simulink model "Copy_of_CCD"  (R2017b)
settings: Solver=FixedStepDiscrete  StartTime=0.0  StopTime=10.0  FixedStep=0.01  RelTol=1e-3  EnableMultiTasking=on
undefined symbols (not defined in the file): ASWTYPE_FALSE, ASWTYPE_TRUE, CcCCD_DrvDiagtCnf_ms, CcCCD_DrvVoltHiVal_mV, CcCCD_DrvVoltLoVal_mV, CcCCD_KL30CVoltCnf_ms, CcCCD_KL30CVoltHiLmt_mV, CcCCD_KL30CVoltLoLmt_mV, CCD_RUNTIME_MS, Enum_CCDLSDState, Enum_UDSAreaSel
libraries: AIWAYS_Powertrain_BMS_lib x38
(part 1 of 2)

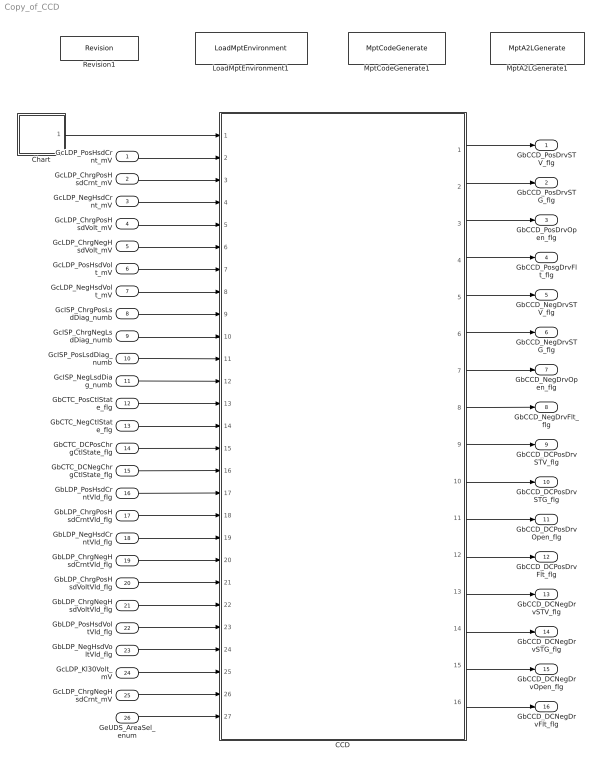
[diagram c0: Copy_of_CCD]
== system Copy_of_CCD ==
  GcLDP_PosHsdCrnt_mV : Inport
  GcLDP_ChrgPosHsdCrnt_mV : Inport  Port=2
  GcLDP_NegHsdCrnt_mV : Inport  Port=3
  GcLDP_ChrgPosHsdVolt_mV : Inport  Port=4
  GcLDP_ChrgNegHsdVolt_mV : Inport  Port=5
  GcLDP_PosHsdVolt_mV : Inport  Port=6
  GcLDP_NegHsdVolt_mV : Inport  Port=7
  GcISP_ChrgPosLsdDiag_numb : Inport  Port=8
  GcISP_ChrgNegLsdDiag_numb : Inport  Port=9
  GcISP_PosLsdDiag_numb : Inport  Port=10
  GcISP_NegLsdDiag_numb : Inport  Port=11
  GbCTC_PosCtlState_flg : Inport  Port=12
  GbCTC_NegCtlState_flg : Inport  Port=13
  GbCTC_DCPosChrgCtlState_flg : Inport  Port=14
  GbCTC_DCNegChrgCtlState_flg : Inport  Port=15
  GbLDP_PosHsdCrntVld_flg : Inport  Port=16
  GbLDP_ChrgPosHsdCrntVld_flg : Inport  Port=17
  GbLDP_NegHsdCrntVld_flg : Inport  Port=18
  GbLDP_ChrgNegHsdCrntVld_flg : Inport  Port=19
  GbLDP_ChrgPosHsdVoltVld_flg : Inport  Port=20
  GbLDP_ChrgNegHsdVoltVld_flg : Inport  Port=21
  GbLDP_PosHsdVoltVld_flg : Inport  Port=22
  GbLDP_NegHsdVoltVld_flg : Inport  Port=23
  GcLDP_Kl30Volt_mV : Inport  Port=24
  GcLDP_ChrgNegHsdCrnt_mV : Inport  Port=25
  GeUDS_AreaSel_enum : Inport  Port=26
  CCD : Subsystem
  Chart : Stateflow chart  TreatAsAtomicUnit=on
  LoadMptEnvironment1 : AIWAYS_Powertrain_BMS_lib/Config/LoadMptEnvironment  ProjectName=Comm  SuppierID=NewPlatformUAES
  MptA2LGenerate1 : AIWAYS_Powertrain_BMS_lib/Config/MptA2LGenerate  SystemSampleTime=-1
  MptCodeGenerate1 : AIWAYS_Powertrain_BMS_lib/Config/MptCodeGenerate  SystemSampleTime=-1
  Revision1 : AIWAYS_Powertrain_BMS_lib/Config/Revision  curVersion='M104C103R102'  newVersion='M104C103R102'
  GbCCD_PosDrvSTV_flg : Outport
  GbCCD_PosDrvSTG_flg : Outport  Port=2
  GbCCD_PosDrvOpen_flg : Outport  Port=3
  GbCCD_PosgDrvFlt_flg : Outport  Port=4
  GbCCD_NegDrvSTV_flg : Outport  Port=5
  GbCCD_NegDrvSTG_flg : Outport  Port=6
  GbCCD_NegDrvOpen_flg : Outport  Port=7
  GbCCD_NegDrvFlt_flg : Outport  Port=8
  GbCCD_DCPosDrvSTV_flg : Outport  Port=9
  GbCCD_DCPosDrvSTG_flg : Outport  Port=10
  GbCCD_DCPosDrvOpen_flg : Outport  Port=11
  GbCCD_DCPosDrvFlt_flg : Outport  Port=12
  GbCCD_DCNegDrvSTV_flg : Outport  Port=13
  GbCCD_DCNegDrvSTG_flg : Outport  Port=14
  GbCCD_DCNegDrvOpen_flg : Outport  Port=15
  GbCCD_DCNegDrvFlt_flg : Outport  Port=16
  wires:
  CCD/1(GbCCD_PosDrvSTV_flg) -> GbCCD_PosDrvSTV_flg/1
  CCD/2(GbCCD_PosDrvSTG_flg) -> GbCCD_PosDrvSTG_flg/1
  CCD/3(GbCCD_PosDrvOpen_flg) -> GbCCD_PosDrvOpen_flg/1
  CCD/5(GbCCD_NegDrvSTV_flg) -> GbCCD_NegDrvSTV_flg/1
  CCD/6(GbCCD_NegDrvSTG_flg) -> GbCCD_NegDrvSTG_flg/1
  CCD/7(GbCCD_NegDrvOpen_flg) -> GbCCD_NegDrvOpen_flg/1
  CCD/9(GbCCD_DCPosDrvSTV_flg) -> GbCCD_DCPosDrvSTV_flg/1
  CCD/10(GbCCD_DCPosDrvSTG_flg) -> GbCCD_DCPosDrvSTG_flg/1
  CCD/11(GbCCD_DCPosDrvOpen_flg) -> GbCCD_DCPosDrvOpen_flg/1
  CCD/13(GbCCD_DCNegDrvSTV_flg) -> GbCCD_DCNegDrvSTV_flg/1
  CCD/14(GbCCD_DCNegDrvSTG_flg) -> GbCCD_DCNegDrvSTG_flg/1
  CCD/15(GbCCD_DCNegDrvOpen_flg) -> GbCCD_DCNegDrvOpen_flg/1
  Chart/1(CCD_CoilDiag_10ms()) -> CCD/1(CCD_CoilDiag_10ms)
  GcLDP_PosHsdCrnt_mV/1 -> CCD/2(GcLDP_PosHsdCrnt_mV)
  GcLDP_ChrgPosHsdCrnt_mV/1 -> CCD/3(GcLDP_ChrgPosHsdCrnt_mV)
  GcLDP_NegHsdCrnt_mV/1 -> CCD/4(GcLDP_NegHsdCrnt_mV)
  GcLDP_ChrgPosHsdVolt_mV/1 -> CCD/5(GcLDP_ChrgPosHsdVolt_mV)
  GcLDP_ChrgNegHsdVolt_mV/1 -> CCD/6(GcLDP_ChrgNegHsdVolt_mV)
  GcLDP_PosHsdVolt_mV/1 -> CCD/7(GcLDP_PosHsdVolt_mV)
  GcLDP_NegHsdVolt_mV/1 -> CCD/8(GcLDP_NegHsdVolt_mV)
  GcISP_ChrgPosLsdDiag_numb/1 -> CCD/9(GcISP_ChrgPosLsdDiag_numb)
  GcISP_ChrgNegLsdDiag_numb/1 -> CCD/10(GcISP_ChrgNegLsdDiag_numb)
  GcISP_PosLsdDiag_numb/1 -> CCD/11(GcISP_PosLsdDiag_numb)
  GcISP_NegLsdDiag_numb/1 -> CCD/12(GcISP_NegLsdDiag_numb)
  GbCTC_PosCtlState_flg/1 -> CCD/13(GbCTC_PosCtlState_flg)
  GbCTC_NegCtlState_flg/1 -> CCD/14(GbCTC_NegCtlState_flg)
  GbCTC_DCPosChrgCtlState_flg/1 -> CCD/15(GbCTC_DCPosChrgCtlState_flg)
  GbCTC_DCNegChrgCtlState_flg/1 -> CCD/16(GbCTC_DCNegChrgCtlState_flg)
  GbLDP_PosHsdCrntVld_flg/1 -> CCD/17(GbLDP_PosHsdCrntVld_flg)
  GbLDP_ChrgPosHsdCrntVld_flg/1 -> CCD/18(GbLDP_ChrgPosHsdCrntVld_flg)
  GbLDP_NegHsdCrntVld_flg/1 -> CCD/19(GbLDP_NegHsdCrntVld_flg)
  GbLDP_ChrgNegHsdCrntVld_flg/1 -> CCD/20(GbLDP_ChrgNegHsdCrntVld_flg)
  GbLDP_ChrgPosHsdVoltVld_flg/1 -> CCD/21(GbLDP_ChrgPosHsdVoltVld_flg)
  GbLDP_ChrgNegHsdVoltVld_flg/1 -> CCD/22(GbLDP_ChrgNegHsdVoltVld_flg)
  GbLDP_PosHsdVoltVld_flg/1 -> CCD/23(GbLDP_PosHsdVoltVld_flg)
  GbLDP_NegHsdVoltVld_flg/1 -> CCD/24(GbLDP_NegHsdVoltVld_flg)
  GcLDP_Kl30Volt_mV/1 -> CCD/25(GcLDP_Kl30Volt_mV)
  GcLDP_ChrgNegHsdCrnt_mV/1 -> CCD/26(GcLDP_ChrgNegHsdCrnt_mV)
  CCD/4(GbCCD_PosgDrvFlt_flg) -> GbCCD_PosgDrvFlt_flg/1
  CCD/8(GbCCD_NegDrvFlt_flg) -> GbCCD_NegDrvFlt_flg/1
  CCD/12(GbCCD_DCPosDrvFlt_flg) -> GbCCD_DCPosDrvFlt_flg/1
  CCD/16(GbCCD_DCNegDrvFlt_flg) -> GbCCD_DCNegDrvFlt_flg/1
  GeUDS_AreaSel_enum/1 -> CCD/27(GeUDS_AreaSel_enum)

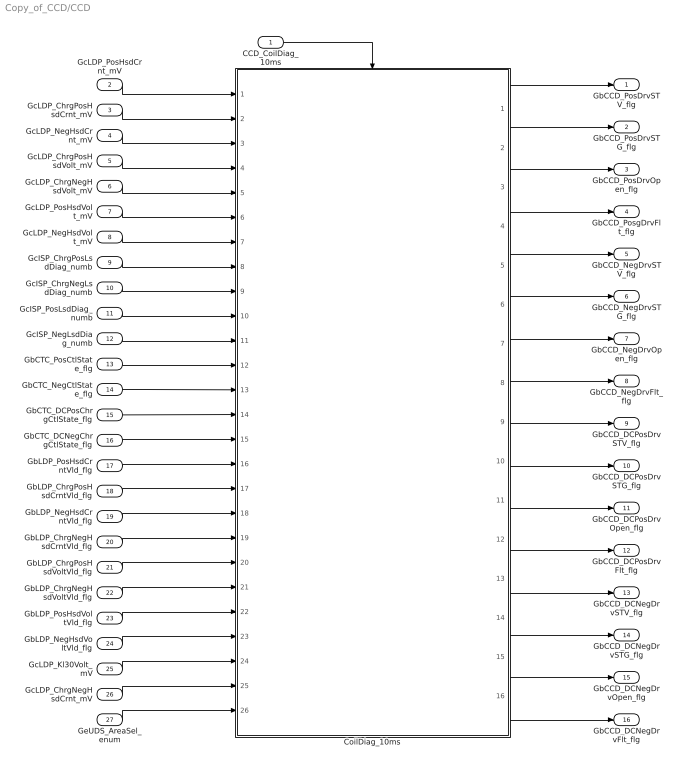
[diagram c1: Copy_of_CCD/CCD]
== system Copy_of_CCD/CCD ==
  CCD_CoilDiag_10ms : Inport
  GcLDP_PosHsdCrnt_mV : Inport  Port=2
  GcLDP_ChrgPosHsdCrnt_mV : Inport  Port=3
  GcLDP_NegHsdCrnt_mV : Inport  Port=4
  GcLDP_ChrgPosHsdVolt_mV : Inport  Port=5
  GcLDP_ChrgNegHsdVolt_mV : Inport  Port=6
  GcLDP_PosHsdVolt_mV : Inport  Port=7
  GcLDP_NegHsdVolt_mV : Inport  Port=8
  GcISP_ChrgPosLsdDiag_numb : Inport  Port=9
  GcISP_ChrgNegLsdDiag_numb : Inport  Port=10
  GcISP_PosLsdDiag_numb : Inport  Port=11
  GcISP_NegLsdDiag_numb : Inport  Port=12
  GbCTC_PosCtlState_flg : Inport  Port=13
  GbCTC_NegCtlState_flg : Inport  Port=14
  GbCTC_DCPosChrgCtlState_flg : Inport  Port=15
  GbCTC_DCNegChrgCtlState_flg : Inport  Port=16
  GbLDP_PosHsdCrntVld_flg : Inport  Port=17
  GbLDP_ChrgPosHsdCrntVld_flg : Inport  Port=18
  GbLDP_NegHsdCrntVld_flg : Inport  Port=19
  GbLDP_ChrgNegHsdCrntVld_flg : Inport  Port=20
  GbLDP_ChrgPosHsdVoltVld_flg : Inport  Port=21
  GbLDP_ChrgNegHsdVoltVld_flg : Inport  Port=22
  GbLDP_PosHsdVoltVld_flg : Inport  Port=23
  GbLDP_NegHsdVoltVld_flg : Inport  Port=24
  GcLDP_Kl30Volt_mV : Inport  Port=25
  GcLDP_ChrgNegHsdCrnt_mV : Inport  Port=26
  GeUDS_AreaSel_enum : Inport  Port=27
  CoilDiag_10ms : Subsystem
  GbCCD_PosDrvSTV_flg : Outport
  GbCCD_PosDrvSTG_flg : Outport  Port=2
  GbCCD_PosDrvOpen_flg : Outport  Port=3
  GbCCD_PosgDrvFlt_flg : Outport  Port=4
  GbCCD_NegDrvSTV_flg : Outport  Port=5
  GbCCD_NegDrvSTG_flg : Outport  Port=6
  GbCCD_NegDrvOpen_flg : Outport  Port=7
  GbCCD_NegDrvFlt_flg : Outport  Port=8
  GbCCD_DCPosDrvSTV_flg : Outport  Port=9
  GbCCD_DCPosDrvSTG_flg : Outport  Port=10
  GbCCD_DCPosDrvOpen_flg : Outport  Port=11
  GbCCD_DCPosDrvFlt_flg : Outport  Port=12
  GbCCD_DCNegDrvSTV_flg : Outport  Port=13
  GbCCD_DCNegDrvSTG_flg : Outport  Port=14
  GbCCD_DCNegDrvOpen_flg : Outport  Port=15
  GbCCD_DCNegDrvFlt_flg : Outport  Port=16
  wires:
  CCD_CoilDiag_10ms/1 -> CoilDiag_10ms/Trigger
  GcLDP_NegHsdVolt_mV/1 -> CoilDiag_10ms/7(GcLDP_NegHsdVolt_mV)
  GcISP_ChrgNegLsdDiag_numb/1 -> CoilDiag_10ms/9(GcISP_ChrgNegLsdDiag_numb)
  GbCTC_PosCtlState_flg/1 -> CoilDiag_10ms/12(GbCTC_PosCtlState_flg)
  CoilDiag_10ms/9(GbCCD_DCPosDrvSTV_flg) -> GbCCD_DCPosDrvSTV_flg/1
  CoilDiag_10ms/13(GbCCD_DCNegDrvSTV_flg) -> GbCCD_DCNegDrvSTV_flg/1
  GcLDP_PosHsdVolt_mV/1 -> CoilDiag_10ms/6(GcLDP_PosHsdVolt_mV)
  CoilDiag_10ms/7(GbCCD_NegDrvOpen_flg) -> GbCCD_NegDrvOpen_flg/1
  CoilDiag_10ms/2(GbCCD_PosDrvSTG_flg) -> GbCCD_PosDrvSTG_flg/1
  GbLDP_NegHsdVoltVld_flg/1 -> CoilDiag_10ms/23(GbLDP_NegHsdVoltVld_flg)
  CoilDiag_10ms/6(GbCCD_NegDrvSTG_flg) -> GbCCD_NegDrvSTG_flg/1
  GbLDP_PosHsdCrntVld_flg/1 -> CoilDiag_10ms/16(GbLDP_PosHsdCrntVld_flg)
  GbLDP_ChrgNegHsdVoltVld_flg/1 -> CoilDiag_10ms/21(GbLDP_ChrgNegHsdVoltVld_flg)
  GbLDP_NegHsdCrntVld_flg/1 -> CoilDiag_10ms/18(GbLDP_NegHsdCrntVld_flg)
  CoilDiag_10ms/3(GbCCD_PosDrvOpen_flg) -> GbCCD_PosDrvOpen_flg/1
  GbLDP_ChrgPosHsdCrntVld_flg/1 -> CoilDiag_10ms/17(GbLDP_ChrgPosHsdCrntVld_flg)
  CoilDiag_10ms/1(GbCCD_PosDrvSTV_flg) -> GbCCD_PosDrvSTV_flg/1
  GbLDP_ChrgNegHsdCrntVld_flg/1 -> CoilDiag_10ms/19(GbLDP_ChrgNegHsdCrntVld_flg)
  CoilDiag_10ms/15(GbCCD_DCNegDrvOpen_flg) -> GbCCD_DCNegDrvOpen_flg/1
  GbLDP_PosHsdVoltVld_flg/1 -> CoilDiag_10ms/22(GbLDP_PosHsdVoltVld_flg)
  GbLDP_ChrgPosHsdVoltVld_flg/1 -> CoilDiag_10ms/20(GbLDP_ChrgPosHsdVoltVld_flg)
  CoilDiag_10ms/11(GbCCD_DCPosDrvOpen_flg) -> GbCCD_DCPosDrvOpen_flg/1
  CoilDiag_10ms/14(GbCCD_DCNegDrvSTG_flg) -> GbCCD_DCNegDrvSTG_flg/1
  GcISP_NegLsdDiag_numb/1 -> CoilDiag_10ms/11(GcISP_NegLsdDiag_numb)
  GbCTC_DCPosChrgCtlState_flg/1 -> CoilDiag_10ms/14(GbCTC_DCPosChrgCtlState_flg)
  GcISP_ChrgPosLsdDiag_numb/1 -> CoilDiag_10ms/8(GcISP_ChrgPosLsdDiag_numb)
  GcLDP_NegHsdCrnt_mV/1 -> CoilDiag_10ms/3(GcLDP_NegHsdCrnt_mV)
  GcLDP_PosHsdCrnt_mV/1 -> CoilDiag_10ms/1(GcLDP_PosHsdCrnt_mV)
  GcLDP_ChrgNegHsdVolt_mV/1 -> CoilDiag_10ms/5(GcLDP_ChrgNegHsdVolt_mV)
  GcISP_PosLsdDiag_numb/1 -> CoilDiag_10ms/10(GcISP_PosLsdDiag_numb)
  GcLDP_ChrgPosHsdCrnt_mV/1 -> CoilDiag_10ms/2(GcLDP_ChrgPosHsdCrnt_mV)
  GcLDP_ChrgPosHsdVolt_mV/1 -> CoilDiag_10ms/4(GcLDP_ChrgPosHsdVolt_mV)
  GbCTC_DCNegChrgCtlState_flg/1 -> CoilDiag_10ms/15(GbCTC_DCNegChrgCtlState_flg)
  GbCTC_NegCtlState_flg/1 -> CoilDiag_10ms/13(GbCTC_NegCtlState_flg)
  CoilDiag_10ms/5(GbCCD_NegDrvSTV_flg) -> GbCCD_NegDrvSTV_flg/1
  CoilDiag_10ms/10(GbCCD_DCPosDrvSTG_flg) -> GbCCD_DCPosDrvSTG_flg/1
  GcLDP_Kl30Volt_mV/1 -> CoilDiag_10ms/24(GcLDP_Kl30Volt_mV)
  GcLDP_ChrgNegHsdCrnt_mV/1 -> CoilDiag_10ms/25(GcLDP_ChrgNegHsdCrnt_mV)
  CoilDiag_10ms/4(GbCCD_PosgDrvFlt_flg) -> GbCCD_PosgDrvFlt_flg/1
  CoilDiag_10ms/8(GbCCD_NegDrvFlt_flg) -> GbCCD_NegDrvFlt_flg/1
  CoilDiag_10ms/12(GbCCD_DCPosDrvFlt_flg) -> GbCCD_DCPosDrvFlt_flg/1
  CoilDiag_10ms/16(GbCCD_DCNegDrvFlt_flg) -> GbCCD_DCNegDrvFlt_flg/1
  GeUDS_AreaSel_enum/1 -> CoilDiag_10ms/26(GeUDS_AreaSel_enum)

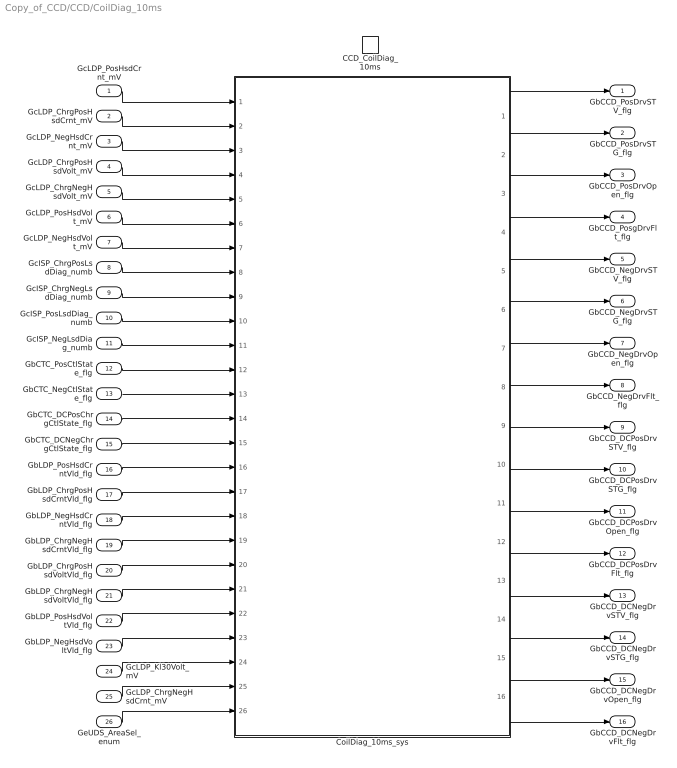
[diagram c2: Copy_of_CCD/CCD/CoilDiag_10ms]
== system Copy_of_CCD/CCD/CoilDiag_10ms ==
  GcLDP_PosHsdCrnt_mV : Inport
  GcLDP_ChrgPosHsdCrnt_mV : Inport  Port=2
  GcLDP_NegHsdCrnt_mV : Inport  Port=3
  GcLDP_ChrgPosHsdVolt_mV : Inport  Port=4
  GcLDP_ChrgNegHsdVolt_mV : Inport  Port=5
  GcLDP_PosHsdVolt_mV : Inport  Port=6
  GcLDP_NegHsdVolt_mV : Inport  Port=7
  GcISP_ChrgPosLsdDiag_numb : Inport  Port=8
  GcISP_ChrgNegLsdDiag_numb : Inport  Port=9
  GcISP_PosLsdDiag_numb : Inport  Port=10
  GcISP_NegLsdDiag_numb : Inport  Port=11
  GbCTC_PosCtlState_flg : Inport  Port=12
  GbCTC_NegCtlState_flg : Inport  Port=13
  GbCTC_DCPosChrgCtlState_flg : Inport  Port=14
  GbCTC_DCNegChrgCtlState_flg : Inport  Port=15
  GbLDP_PosHsdCrntVld_flg : Inport  Port=16
  GbLDP_ChrgPosHsdCrntVld_flg : Inport  Port=17
  GbLDP_NegHsdCrntVld_flg : Inport  Port=18
  GbLDP_ChrgNegHsdCrntVld_flg : Inport  Port=19
  GbLDP_ChrgPosHsdVoltVld_flg : Inport  Port=20
  GbLDP_ChrgNegHsdVoltVld_flg : Inport  Port=21
  GbLDP_PosHsdVoltVld_flg : Inport  Port=22
  GbLDP_NegHsdVoltVld_flg : Inport  Port=23
  GcLDP_Kl30Volt_mV : Inport  Port=24
  GcLDP_ChrgNegHsdCrnt_mV : Inport  Port=25
  GeUDS_AreaSel_enum : Inport  Port=26
  CCD_CoilDiag_10ms : TriggerPort  TriggerType=function-call  VariantControl=(inherit)
  CoilDiag_10ms_sys : Subsystem
  GbCCD_PosDrvSTV_flg : Outport
  GbCCD_PosDrvSTG_flg : Outport  Port=2
  GbCCD_PosDrvOpen_flg : Outport  Port=3
  GbCCD_PosgDrvFlt_flg : Outport  Port=4
  GbCCD_NegDrvSTV_flg : Outport  Port=5
  GbCCD_NegDrvSTG_flg : Outport  Port=6
  GbCCD_NegDrvOpen_flg : Outport  Port=7
  GbCCD_NegDrvFlt_flg : Outport  Port=8
  GbCCD_DCPosDrvSTV_flg : Outport  Port=9
  GbCCD_DCPosDrvSTG_flg : Outport  Port=10
  GbCCD_DCPosDrvOpen_flg : Outport  Port=11
  GbCCD_DCPosDrvFlt_flg : Outport  Port=12
  GbCCD_DCNegDrvSTV_flg : Outport  Port=13
  GbCCD_DCNegDrvSTG_flg : Outport  Port=14
  GbCCD_DCNegDrvOpen_flg : Outport  Port=15
  GbCCD_DCNegDrvFlt_flg : Outport  Port=16
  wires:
  GcLDP_PosHsdCrnt_mV/1 -> CoilDiag_10ms_sys/1(GcLDP_PosHsdCrnt_mV)
  GcLDP_ChrgPosHsdCrnt_mV/1 -> CoilDiag_10ms_sys/2(GcLDP_ChrgPosHsdCrnt_mV)
  GcLDP_NegHsdCrnt_mV/1 -> CoilDiag_10ms_sys/3(GcLDP_NegHsdCrnt_mV)
  GcLDP_ChrgPosHsdVolt_mV/1 -> CoilDiag_10ms_sys/4(GcLDP_ChrgPosHsdVolt_mV)
  GcLDP_ChrgNegHsdVolt_mV/1 -> CoilDiag_10ms_sys/5(GcLDP_ChrgNegHsdVolt_mV)
  GcLDP_PosHsdVolt_mV/1 -> CoilDiag_10ms_sys/6(GcLDP_PosHsdVolt_mV)
  GcLDP_NegHsdVolt_mV/1 -> CoilDiag_10ms_sys/7(GcLDP_NegHsdVolt_mV)
  GcISP_ChrgPosLsdDiag_numb/1 -> CoilDiag_10ms_sys/8(GcISP_ChrgPosLsdDiag_numb)
  GcISP_ChrgNegLsdDiag_numb/1 -> CoilDiag_10ms_sys/9(GcISP_ChrgNegLsdDiag_numb)
  GcISP_PosLsdDiag_numb/1 -> CoilDiag_10ms_sys/10(GcISP_PosLsdDiag_numb)
  GcISP_NegLsdDiag_numb/1 -> CoilDiag_10ms_sys/11(GcISP_NegLsdDiag_numb)
  GbCTC_PosCtlState_flg/1 -> CoilDiag_10ms_sys/12(GbCTC_PosCtlState_flg)
  GbCTC_NegCtlState_flg/1 -> CoilDiag_10ms_sys/13(GbCTC_NegCtlState_flg)
  GbCTC_DCPosChrgCtlState_flg/1 -> CoilDiag_10ms_sys/14(GbCTC_DCPosChrgCtlState_flg)
  GbCTC_DCNegChrgCtlState_flg/1 -> CoilDiag_10ms_sys/15(GbCTC_DCNegChrgCtlState_flg)
  GbLDP_ChrgPosHsdCrntVld_flg/1 -> CoilDiag_10ms_sys/17(GbLDP_ChrgPosHsdCrntVld_flg)
  GbLDP_PosHsdCrntVld_flg/1 -> CoilDiag_10ms_sys/16(GbLDP_PosHsdCrntVld_flg)
  GbLDP_NegHsdCrntVld_flg/1 -> CoilDiag_10ms_sys/18(GbLDP_NegHsdCrntVld_flg)
  GbLDP_ChrgNegHsdCrntVld_flg/1 -> CoilDiag_10ms_sys/19(GbLDP_ChrgNegHsdCrntVld_flg)
  GbLDP_ChrgPosHsdVoltVld_flg/1 -> CoilDiag_10ms_sys/20(GbLDP_ChrgPosHsdVoltVld_flg)
  GbLDP_ChrgNegHsdVoltVld_flg/1 -> CoilDiag_10ms_sys/21(GbLDP_ChrgNegHsdVoltVld_flg)
  GbLDP_PosHsdVoltVld_flg/1 -> CoilDiag_10ms_sys/22(GbLDP_PosHsdVoltVld_flg)
  GbLDP_NegHsdVoltVld_flg/1 -> CoilDiag_10ms_sys/23(GbLDP_NegHsdVoltVld_flg)
  CoilDiag_10ms_sys/15(GbCCD_DCNegDrvOpen_flg) -> GbCCD_DCNegDrvOpen_flg/1
  CoilDiag_10ms_sys/1(GbCCD_PosDrvSTV_flg) -> GbCCD_PosDrvSTV_flg/1
  CoilDiag_10ms_sys/2(GbCCD_PosDrvSTG_flg) -> GbCCD_PosDrvSTG_flg/1
  CoilDiag_10ms_sys/3(GbCCD_PosDrvOpen_flg) -> GbCCD_PosDrvOpen_flg/1
  CoilDiag_10ms_sys/5(GbCCD_NegDrvSTV_flg) -> GbCCD_NegDrvSTV_flg/1
  CoilDiag_10ms_sys/6(GbCCD_NegDrvSTG_flg) -> GbCCD_NegDrvSTG_flg/1
  CoilDiag_10ms_sys/7(GbCCD_NegDrvOpen_flg) -> GbCCD_NegDrvOpen_flg/1
  CoilDiag_10ms_sys/9(GbCCD_DCPosDrvSTV_flg) -> GbCCD_DCPosDrvSTV_flg/1
  CoilDiag_10ms_sys/10(GbCCD_DCPosDrvSTG_flg) -> GbCCD_DCPosDrvSTG_flg/1
  CoilDiag_10ms_sys/11(GbCCD_DCPosDrvOpen_flg) -> GbCCD_DCPosDrvOpen_flg/1
  CoilDiag_10ms_sys/13(GbCCD_DCNegDrvSTV_flg) -> GbCCD_DCNegDrvSTV_flg/1
  CoilDiag_10ms_sys/14(GbCCD_DCNegDrvSTG_flg) -> GbCCD_DCNegDrvSTG_flg/1
  GcLDP_Kl30Volt_mV/1 -> CoilDiag_10ms_sys/24(GcLDP_Kl30Volt_mV)
  GcLDP_ChrgNegHsdCrnt_mV/1 -> CoilDiag_10ms_sys/25(GcLDP_ChrgNegHsdCrnt_mV)
  CoilDiag_10ms_sys/4(GbCCD_PosgDrvFlt_flg) -> GbCCD_PosgDrvFlt_flg/1
  CoilDiag_10ms_sys/8(GbCCD_NegDrvFlt_flg) -> GbCCD_NegDrvFlt_flg/1
  CoilDiag_10ms_sys/12(GbCCD_DCPosDrvFlt_flg) -> GbCCD_DCPosDrvFlt_flg/1
  CoilDiag_10ms_sys/16(GbCCD_DCNegDrvFlt_flg) -> GbCCD_DCNegDrvFlt_flg/1
  GeUDS_AreaSel_enum/1 -> CoilDiag_10ms_sys/26(GeUDS_AreaSel_enum)

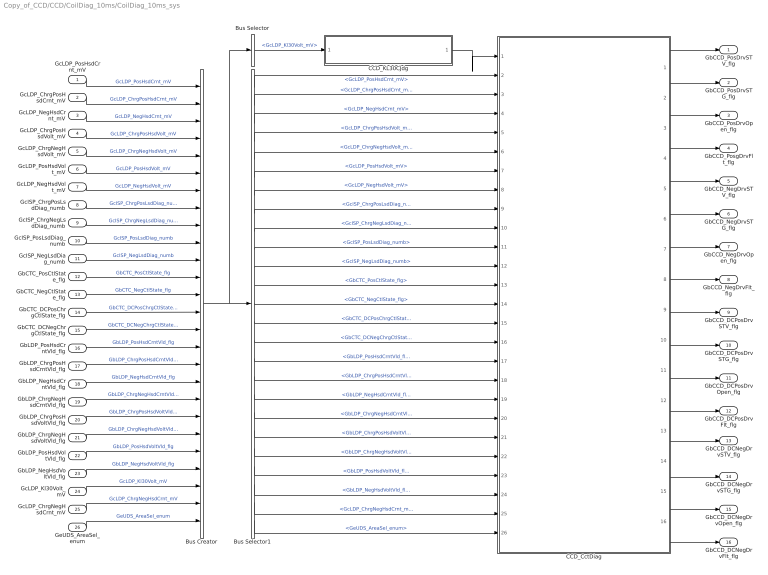
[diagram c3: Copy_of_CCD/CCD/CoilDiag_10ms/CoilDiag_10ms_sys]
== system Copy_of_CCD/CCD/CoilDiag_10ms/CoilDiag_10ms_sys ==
  GcLDP_PosHsdCrnt_mV : Inport
  GcLDP_ChrgPosHsdCrnt_mV : Inport  Port=2
  GcLDP_NegHsdCrnt_mV : Inport  Port=3
  GcLDP_ChrgPosHsdVolt_mV : Inport  Port=4
  GcLDP_ChrgNegHsdVolt_mV : Inport  Port=5
  GcLDP_PosHsdVolt_mV : Inport  Port=6
  GcLDP_NegHsdVolt_mV : Inport  Port=7
  GcISP_ChrgPosLsdDiag_numb : Inport  Port=8
  GcISP_ChrgNegLsdDiag_numb : Inport  Port=9
  GcISP_PosLsdDiag_numb : Inport  Port=10
  GcISP_NegLsdDiag_numb : Inport  Port=11
  GbCTC_PosCtlState_flg : Inport  Port=12
  GbCTC_NegCtlState_flg : Inport  Port=13
  GbCTC_DCPosChrgCtlState_flg : Inport  Port=14
  GbCTC_DCNegChrgCtlState_flg : Inport  Port=15
  GbLDP_PosHsdCrntVld_flg : Inport  Port=16
  GbLDP_ChrgPosHsdCrntVld_flg : Inport  Port=17
  GbLDP_NegHsdCrntVld_flg : Inport  Port=18
  GbLDP_ChrgNegHsdCrntVld_flg : Inport  Port=19
  GbLDP_ChrgPosHsdVoltVld_flg : Inport  Port=20
  GbLDP_ChrgNegHsdVoltVld_flg : Inport  Port=21
  GbLDP_PosHsdVoltVld_flg : Inport  Port=22
  GbLDP_NegHsdVoltVld_flg : Inport  Port=23
  GcLDP_Kl30Volt_mV : Inport  Port=24
  GcLDP_ChrgNegHsdCrnt_mV : Inport  Port=25
  GeUDS_AreaSel_enum : Inport  Port=26
  Bus Creator : BusCreator  Inputs=26
  Bus Selector : BusSelector  OutputSignals=GcLDP_Kl30Volt_mV
  Bus Selector1 : BusSelector  OutputSignals=GcLDP_PosHsdCrnt_mV,GcLDP_ChrgPosHsdCrnt_mV,GcLDP_NegHsdCrnt_mV,GcLDP_ChrgPosHsdVolt_mV,GcLDP_ChrgNegHsdVolt_mV,GcLDP_PosHsdVolt_mV,GcLDP_NegHsdVolt_mV,GcISP_ChrgPosLsdDiag_numb,GcISP_ChrgNegLsdDiag_numb,GcISP_PosLsdDiag_numb,GcISP_NegLsdDiag_numb,GbCTC_PosCtlState_flg,GbCTC_NegCtlState_flg,GbCTC_DCPosChrgCtlState_flg,GbCTC_DCNegChrgCtlState_flg,GbLDP_PosHsdCrntVld_flg,GbLDP_ChrgPosHsdCrntVld_flg,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
  CCD_CctDiag : Subsystem
  CCD_KL30CJdg : Subsystem
  GbCCD_PosDrvSTV_flg : Outport
  GbCCD_PosDrvSTG_flg : Outport  Port=2
  GbCCD_PosDrvOpen_flg : Outport  Port=3
  GbCCD_PosgDrvFlt_flg : Outport  Port=4
  GbCCD_NegDrvSTV_flg : Outport  Port=5
  GbCCD_NegDrvSTG_flg : Outport  Port=6
  GbCCD_NegDrvOpen_flg : Outport  Port=7
  GbCCD_NegDrvFlt_flg : Outport  Port=8
  GbCCD_DCPosDrvSTV_flg : Outport  Port=9
  GbCCD_DCPosDrvSTG_flg : Outport  Port=10
  GbCCD_DCPosDrvOpen_flg : Outport  Port=11
  GbCCD_DCPosDrvFlt_flg : Outport  Port=12
  GbCCD_DCNegDrvSTV_flg : Outport  Port=13
  GbCCD_DCNegDrvSTG_flg : Outport  Port=14
  GbCCD_DCNegDrvOpen_flg : Outport  Port=15
  GbCCD_DCNegDrvFlt_flg : Outport  Port=16
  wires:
  GcLDP_PosHsdCrnt_mV/1 -> Bus Creator/1  "GcLDP_PosHsdCrnt_mV"
  GcLDP_ChrgPosHsdCrnt_mV/1 -> Bus Creator/2  "GcLDP_ChrgPosHsdCrnt_mV"
  GcLDP_NegHsdCrnt_mV/1 -> Bus Creator/3  "GcLDP_NegHsdCrnt_mV"
  GcLDP_ChrgPosHsdVolt_mV/1 -> Bus Creator/4  "GcLDP_ChrgPosHsdVolt_mV"
  GcLDP_ChrgNegHsdVolt_mV/1 -> Bus Creator/5  "GcLDP_ChrgNegHsdVolt_mV"
  GcLDP_PosHsdVolt_mV/1 -> Bus Creator/6  "GcLDP_PosHsdVolt_mV"
  GcLDP_NegHsdVolt_mV/1 -> Bus Creator/7  "GcLDP_NegHsdVolt_mV"
  GcISP_ChrgPosLsdDiag_numb/1 -> Bus Creator/8  "GcISP_ChrgPosLsdDiag_numb"
  GcISP_ChrgNegLsdDiag_numb/1 -> Bus Creator/9  "GcISP_ChrgNegLsdDiag_numb"
  GcISP_PosLsdDiag_numb/1 -> Bus Creator/10  "GcISP_PosLsdDiag_numb"
  GcISP_NegLsdDiag_numb/1 -> Bus Creator/11  "GcISP_NegLsdDiag_numb"
  GbCTC_PosCtlState_flg/1 -> Bus Creator/12  "GbCTC_PosCtlState_flg"
  GbCTC_NegCtlState_flg/1 -> Bus Creator/13  "GbCTC_NegCtlState_flg"
  GbCTC_DCPosChrgCtlState_flg/1 -> Bus Creator/14  "GbCTC_DCPosChrgCtlState_flg"
  GbCTC_DCNegChrgCtlState_flg/1 -> Bus Creator/15  "GbCTC_DCNegChrgCtlState_flg"
  GbLDP_PosHsdCrntVld_flg/1 -> Bus Creator/16  "GbLDP_PosHsdCrntVld_flg"
  GbLDP_ChrgPosHsdCrntVld_flg/1 -> Bus Creator/17  "GbLDP_ChrgPosHsdCrntVld_flg"
  GbLDP_NegHsdCrntVld_flg/1 -> Bus Creator/18  "GbLDP_NegHsdCrntVld_flg"
  GbLDP_ChrgNegHsdCrntVld_flg/1 -> Bus Creator/19  "GbLDP_ChrgNegHsdCrntVld_flg"
  GbLDP_ChrgPosHsdVoltVld_flg/1 -> Bus Creator/20  "GbLDP_ChrgPosHsdVoltVld_flg"
  GbLDP_ChrgNegHsdVoltVld_flg/1 -> Bus Creator/21  "GbLDP_ChrgNegHsdVoltVld_flg"
  GbLDP_PosHsdVoltVld_flg/1 -> Bus Creator/22  "GbLDP_PosHsdVoltVld_flg"
  GbLDP_NegHsdVoltVld_flg/1 -> Bus Creator/23  "GbLDP_NegHsdVoltVld_flg"
  GcLDP_Kl30Volt_mV/1 -> Bus Creator/24  "GcLDP_Kl30Volt_mV"
  Bus Creator/1 -> Bus Selector1/1, Bus Selector/1
  Bus Selector/1 -> CCD_KL30CJdg/1(GcLDP_Kl30Volt_mV)  "<GcLDP_Kl30Volt_mV>"
  CCD_KL30CJdg/1(LbCCD_CCDDiag_flg) -> CCD_CctDiag/1(LbCCD_CCDDiag_flg)
  Bus Selector1/1 -> CCD_CctDiag/2(GcLDP_PosHsdCrnt_mV)  "<GcLDP_PosHsdCrnt_mV>"
  Bus Selector1/2 -> CCD_CctDiag/3(GcLDP_ChrgPosHsdCrnt_mV)  "<GcLDP_ChrgPosHsdCrnt_mV>"
  Bus Selector1/3 -> CCD_CctDiag/4(GcLDP_NegHsdCrnt_mV)  "<GcLDP_NegHsdCrnt_mV>"
  Bus Selector1/4 -> CCD_CctDiag/5(GcLDP_ChrgPosHsdVolt_mV)  "<GcLDP_ChrgPosHsdVolt_mV>"
  Bus Selector1/5 -> CCD_CctDiag/6(GcLDP_ChrgNegHsdVolt_mV)  "<GcLDP_ChrgNegHsdVolt_mV>"
  Bus Selector1/6 -> CCD_CctDiag/7(GcLDP_PosHsdVolt_mV)  "<GcLDP_PosHsdVolt_mV>"
  Bus Selector1/7 -> CCD_CctDiag/8(GcLDP_NegHsdVolt_mV)  "<GcLDP_NegHsdVolt_mV>"
  Bus Selector1/8 -> CCD_CctDiag/9(GcISP_ChrgPosLsdDiag_numb)  "<GcISP_ChrgPosLsdDiag_numb>"
  Bus Selector1/9 -> CCD_CctDiag/10(GcISP_ChrgNegLsdDiag_numb)  "<GcISP_ChrgNegLsdDiag_numb>"
  Bus Selector1/10 -> CCD_CctDiag/11(GcISP_PosLsdDiag_numb)  "<GcISP_PosLsdDiag_numb>"
  Bus Selector1/11 -> CCD_CctDiag/12(GcISP_NegLsdDiag_numb)  "<GcISP_NegLsdDiag_numb>"
  Bus Selector1/12 -> CCD_CctDiag/13(GbCTC_PosCtlState_flg)  "<GbCTC_PosCtlState_flg>"
  Bus Selector1/13 -> CCD_CctDiag/14(GbCTC_NegCtlState_flg)  "<GbCTC_NegCtlState_flg>"
  Bus Selector1/14 -> CCD_CctDiag/15(GbCTC_DCPosChrgCtlState_flg)  "<GbCTC_DCPosChrgCtlState_flg>"
  Bus Selector1/15 -> CCD_CctDiag/16(GbCTC_DCNegChrgCtlState_flg)  "<GbCTC_DCNegChrgCtlState_flg>"
  Bus Selector1/16 -> CCD_CctDiag/17(GbLDP_PosHsdCrntVld_flg)  "<GbLDP_PosHsdCrntVld_flg>"
  Bus Selector1/17 -> CCD_CctDiag/18(GbLDP_ChrgPosHsdCrntVld_flg)  "<GbLDP_ChrgPosHsdCrntVld_flg>"
  Bus Selector1/18 -> CCD_CctDiag/19(GbLDP_NegHsdCrntVld_flg)  "<GbLDP_NegHsdCrntVld_flg>"
  Bus Selector1/19 -> CCD_CctDiag/20(GbLDP_ChrgNegHsdCrntVld_flg)  "<GbLDP_ChrgNegHsdCrntVld_flg>"
  Bus Selector1/20 -> CCD_CctDiag/21(GbLDP_ChrgPosHsdVoltVld_flg)  "<GbLDP_ChrgPosHsdVoltVld_flg>"
  Bus Selector1/21 -> CCD_CctDiag/22(GbLDP_ChrgNegHsdVoltVld_flg)  "<GbLDP_ChrgNegHsdVoltVld_flg>"
  Bus Selector1/22 -> CCD_CctDiag/23(GbLDP_PosHsdVoltVld_flg)  "<GbLDP_PosHsdVoltVld_flg>"
  Bus Selector1/23 -> CCD_CctDiag/24(GbLDP_NegHsdVoltVld_flg)  "<GbLDP_NegHsdVoltVld_flg>"
  CCD_CctDiag/1(GbCCD_PosDrvSTV_flg) -> GbCCD_PosDrvSTV_flg/1
  CCD_CctDiag/2(GbCCD_PosDrvSTG_flg) -> GbCCD_PosDrvSTG_flg/1
  CCD_CctDiag/3(GbCCD_PosDrvOpen_flg) -> GbCCD_PosDrvOpen_flg/1
  CCD_CctDiag/5(GbCCD_NegDrvSTV_flg) -> GbCCD_NegDrvSTV_flg/1
  CCD_CctDiag/6(GbCCD_NegDrvSTG_flg) -> GbCCD_NegDrvSTG_flg/1
  CCD_CctDiag/7(GbCCD_NegDrvOpen_flg) -> GbCCD_NegDrvOpen_flg/1
  CCD_CctDiag/9(GbCCD_DCPosDrvSTV_flg) -> GbCCD_DCPosDrvSTV_flg/1
  CCD_CctDiag/10(GbCCD_DCPosDrvSTG_flg) -> GbCCD_DCPosDrvSTG_flg/1
  CCD_CctDiag/11(GbCCD_DCPosDrvOpen_flg) -> GbCCD_DCPosDrvOpen_flg/1
  CCD_CctDiag/13(GbCCD_DCNegDrvSTV_flg) -> GbCCD_DCNegDrvSTV_flg/1
  CCD_CctDiag/14(GbCCD_DCNegDrvSTG_flg) -> GbCCD_DCNegDrvSTG_flg/1
  CCD_CctDiag/15(GbCCD_DCNegDrvOpen_flg) -> GbCCD_DCNegDrvOpen_flg/1
  GcLDP_ChrgNegHsdCrnt_mV/1 -> Bus Creator/25  "GcLDP_ChrgNegHsdCrnt_mV"
  Bus Selector1/24 -> CCD_CctDiag/25(GcLDP_ChrgNegHsdCrnt_mV)  "<GcLDP_ChrgNegHsdCrnt_mV>"
  CCD_CctDiag/4(GbCCD_PosgDrvFlt_flg) -> GbCCD_PosgDrvFlt_flg/1
  CCD_CctDiag/8(GbCCD_NegDrvFlt_flg) -> GbCCD_NegDrvFlt_flg/1
  CCD_CctDiag/12(GbCCD_DCPosDrvFlt_flg) -> GbCCD_DCPosDrvFlt_flg/1
  CCD_CctDiag/16(GbCCD_DCNegDrvFlt_flg) -> GbCCD_DCNegDrvFlt_flg/1
  GeUDS_AreaSel_enum/1 -> Bus Creator/26  "GeUDS_AreaSel_enum"
  Bus Selector1/25 -> CCD_CctDiag/26(GeUDS_AreaSel_enum)  "<GeUDS_AreaSel_enum>"

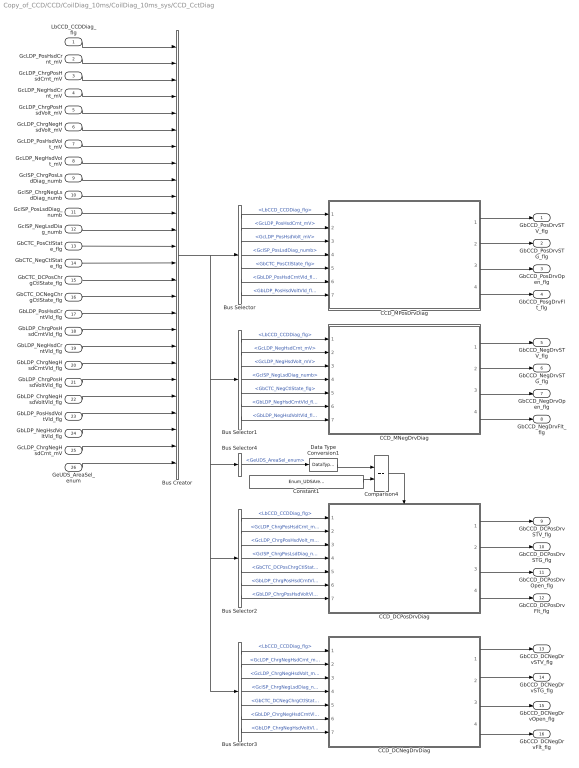
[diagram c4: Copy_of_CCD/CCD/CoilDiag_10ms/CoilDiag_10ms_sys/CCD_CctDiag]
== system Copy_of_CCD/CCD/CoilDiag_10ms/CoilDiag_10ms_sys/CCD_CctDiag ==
  LbCCD_CCDDiag_flg : Inport
  GcLDP_PosHsdCrnt_mV : Inport  Port=2
  GcLDP_ChrgPosHsdCrnt_mV : Inport  Port=3
  GcLDP_NegHsdCrnt_mV : Inport  Port=4
  GcLDP_ChrgPosHsdVolt_mV : Inport  Port=5
  GcLDP_ChrgNegHsdVolt_mV : Inport  Port=6
  GcLDP_PosHsdVolt_mV : Inport  Port=7
  GcLDP_NegHsdVolt_mV : Inport  Port=8
  GcISP_ChrgPosLsdDiag_numb : Inport  Port=9
  GcISP_ChrgNegLsdDiag_numb : Inport  Port=10
  GcISP_PosLsdDiag_numb : Inport  Port=11
  GcISP_NegLsdDiag_numb : Inport  Port=12
  GbCTC_PosCtlState_flg : Inport  Port=13
  GbCTC_NegCtlState_flg : Inport  Port=14
  GbCTC_DCPosChrgCtlState_flg : Inport  Port=15
  GbCTC_DCNegChrgCtlState_flg : Inport  Port=16
  GbLDP_PosHsdCrntVld_flg : Inport  Port=17
  GbLDP_ChrgPosHsdCrntVld_flg : Inport  Port=18
  GbLDP_NegHsdCrntVld_flg : Inport  Port=19
  GbLDP_ChrgNegHsdCrntVld_flg : Inport  Port=20
  GbLDP_ChrgPosHsdVoltVld_flg : Inport  Port=21
  GbLDP_ChrgNegHsdVoltVld_flg : Inport  Port=22
  GbLDP_PosHsdVoltVld_flg : Inport  Port=23
  GbLDP_NegHsdVoltVld_flg : Inport  Port=24
  GcLDP_ChrgNegHsdCrnt_mV : Inport  Port=25
  GeUDS_AreaSel_enum : Inport  Port=26
  Bus Creator : BusCreator  Inputs=26
  Bus Selector : BusSelector  OutputSignals=LbCCD_CCDDiag_flg,GcLDP_PosHsdCrnt_mV,GcLDP_PosHsdVolt_mV,GcISP_PosLsdDiag_numb,GbCTC_PosCtlState_flg,GbLDP_PosHsdCrntVld_flg,GbLDP_PosHsdVoltVld_flg
  Bus Selector1 : BusSelector  OutputSignals=LbCCD_CCDDiag_flg,GcLDP_NegHsdCrnt_mV,GcLDP_NegHsdVolt_mV,GcISP_NegLsdDiag_numb,GbCTC_NegCtlState_flg,GbLDP_NegHsdCrntVld_flg,GbLDP_NegHsdVoltVld_flg
  Bus Selector2 : BusSelector  OutputSignals=LbCCD_CCDDiag_flg,GcLDP_ChrgPosHsdCrnt_mV,GcLDP_ChrgPosHsdVolt_mV,GcISP_ChrgPosLsdDiag_numb,GbCTC_DCPosChrgCtlState_flg,GbLDP_ChrgPosHsdCrntVld_flg,GbLDP_ChrgPosHsdVoltVld_flg
  Bus Selector3 : BusSelector  OutputSignals=LbCCD_CCDDiag_flg,GcLDP_ChrgNegHsdCrnt_mV,GcLDP_ChrgNegHsdVolt_mV,GcISP_ChrgNegLsdDiag_numb,GbCTC_DCNegChrgCtlState_flg,GbLDP_ChrgNegHsdCrntVld_flg,GbLDP_ChrgNegHsdVoltVld_flg
  Bus Selector4 : BusSelector  OutputSignals=GeUDS_AreaSel_enum
  CCD_DCNegDrvDiag : Subsystem
  CCD_DCPosDrvDiag : Subsystem
  CCD_MNegDrvDiag : Subsystem
  CCD_MPosDrvDiag : Subsystem
  Comparison4 : RelationalOperator  Operator===  OutDataTypeStr=boolean
  Constant1 : Constant  Value=Enum_UDSAreaSel.Enum_UDSAreaSel_EU
  Data Type Conversion1 : DataTypeConversion
  GbCCD_PosDrvSTV_flg : Outport
  GbCCD_PosDrvSTG_flg : Outport  Port=2
  GbCCD_PosDrvOpen_flg : Outport  Port=3
  GbCCD_PosgDrvFlt_flg : Outport  Port=4
  GbCCD_NegDrvSTV_flg : Outport  Port=5
  GbCCD_NegDrvSTG_flg : Outport  Port=6
  GbCCD_NegDrvOpen_flg : Outport  Port=7
  GbCCD_NegDrvFlt_flg : Outport  Port=8
  GbCCD_DCPosDrvSTV_flg : Outport  Port=9
  GbCCD_DCPosDrvSTG_flg : Outport  Port=10
  GbCCD_DCPosDrvOpen_flg : Outport  Port=11
  GbCCD_DCPosDrvFlt_flg : Outport  Port=12
  GbCCD_DCNegDrvSTV_flg : Outport  Port=13
  GbCCD_DCNegDrvSTG_flg : Outport  Port=14
  GbCCD_DCNegDrvOpen_flg : Outport  Port=15
  GbCCD_DCNegDrvFlt_flg : Outport  Port=16
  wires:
  Bus Creator/1 -> Bus Selector4/1, Bus Selector3/1, Bus Selector2/1, Bus Selector1/1, Bus Selector/1
  Bus Selector/3 -> CCD_MPosDrvDiag/3(GcLDP_PosHsdVolt_mV)  "<GcLDP_PosHsdVolt_mV>"
  Bus Selector/4 -> CCD_MPosDrvDiag/4(GcISP_PosLsdDiag_numb)  "<GcISP_PosLsdDiag_numb>"
  Bus Selector/7 -> CCD_MPosDrvDiag/7(GbLDP_PosHsdVoltVld_flg)  "<GbLDP_PosHsdVoltVld_flg>"
  Bus Selector/2 -> CCD_MPosDrvDiag/2(GcLDP_PosHsdCrnt_mV)  "<GcLDP_PosHsdCrnt_mV>"
  Bus Selector/5 -> CCD_MPosDrvDiag/5(GbCTC_PosCtlState_flg)  "<GbCTC_PosCtlState_flg>"
  Bus Selector/6 -> CCD_MPosDrvDiag/6(GbLDP_PosHsdCrntVld_flg)  "<GbLDP_PosHsdCrntVld_flg>"
  CCD_MPosDrvDiag/1(GbCCD_PosDrvSTV_flg) -> GbCCD_PosDrvSTV_flg/1
  CCD_MPosDrvDiag/2(GbCCD_PosDrvSTG_flg) -> GbCCD_PosDrvSTG_flg/1
  CCD_MPosDrvDiag/3(GbCCD_PosDrvOpen_flg) -> GbCCD_PosDrvOpen_flg/1
  LbCCD_CCDDiag_flg/1 -> Bus Creator/1
  GcLDP_PosHsdCrnt_mV/1 -> Bus Creator/2
  GcLDP_ChrgPosHsdCrnt_mV/1 -> Bus Creator/3
  GcLDP_NegHsdCrnt_mV/1 -> Bus Creator/4
  GcLDP_ChrgPosHsdVolt_mV/1 -> Bus Creator/5
  GcLDP_ChrgNegHsdVolt_mV/1 -> Bus Creator/6
  GcLDP_PosHsdVolt_mV/1 -> Bus Creator/7
  GcLDP_NegHsdVolt_mV/1 -> Bus Creator/8
  GcISP_ChrgPosLsdDiag_numb/1 -> Bus Creator/9
  GcISP_ChrgNegLsdDiag_numb/1 -> Bus Creator/10
  GcISP_PosLsdDiag_numb/1 -> Bus Creator/11
  GcISP_NegLsdDiag_numb/1 -> Bus Creator/12
  GbCTC_PosCtlState_flg/1 -> Bus Creator/13
  GbCTC_NegCtlState_flg/1 -> Bus Creator/14
  GbCTC_DCPosChrgCtlState_flg/1 -> Bus Creator/15
  GbCTC_DCNegChrgCtlState_flg/1 -> Bus Creator/16
  GbLDP_PosHsdCrntVld_flg/1 -> Bus Creator/17
  GbLDP_ChrgPosHsdCrntVld_flg/1 -> Bus Creator/18
  GbLDP_NegHsdCrntVld_flg/1 -> Bus Creator/19
  GbLDP_ChrgNegHsdCrntVld_flg/1 -> Bus Creator/20
  GbLDP_ChrgPosHsdVoltVld_flg/1 -> Bus Creator/21
  GbLDP_ChrgNegHsdVoltVld_flg/1 -> Bus Creator/22
  GbLDP_PosHsdVoltVld_flg/1 -> Bus Creator/23
  GbLDP_NegHsdVoltVld_flg/1 -> Bus Creator/24
  Bus Selector/1 -> CCD_MPosDrvDiag/1(LbCCD_CCDDiag_flg)  "<LbCCD_CCDDiag_flg>"
  Bus Selector1/1 -> CCD_MNegDrvDiag/1(LbCCD_CCDDiag_flg)  "<LbCCD_CCDDiag_flg>"
  Bus Selector1/2 -> CCD_MNegDrvDiag/2(GcLDP_NegHsdCrnt_mV)  "<GcLDP_NegHsdCrnt_mV>"
  Bus Selector1/3 -> CCD_MNegDrvDiag/3(GcLDP_NegHsdVolt_mV)  "<GcLDP_NegHsdVolt_mV>"
  Bus Selector1/4 -> CCD_MNegDrvDiag/4(GcISP_NegLsdDiag_numb)  "<GcISP_NegLsdDiag_numb>"
  Bus Selector1/5 -> CCD_MNegDrvDiag/5(GbCTC_NegCtlState_flg)  "<GbCTC_NegCtlState_flg>"
  Bus Selector1/6 -> CCD_MNegDrvDiag/6(GbLDP_NegHsdCrntVld_flg)  "<GbLDP_NegHsdCrntVld_flg>"
  Bus Selector1/7 -> CCD_MNegDrvDiag/7(GbLDP_NegHsdVoltVld_flg)  "<GbLDP_NegHsdVoltVld_flg>"
  CCD_MNegDrvDiag/1(GbCCD_NegDrvSTV_flg) -> GbCCD_NegDrvSTV_flg/1
  CCD_MNegDrvDiag/3(GbCCD_NegDrvOpen_flg) -> GbCCD_NegDrvOpen_flg/1
  CCD_MNegDrvDiag/2(GbCCD_NegDrvSTG_flg) -> GbCCD_NegDrvSTG_flg/1
  Bus Selector2/1 -> CCD_DCPosDrvDiag/1(LbCCD_CCDDiag_flg)  "<LbCCD_CCDDiag_flg>"
  Bus Selector2/2 -> CCD_DCPosDrvDiag/2(GcLDP_ChrgPosHsdCrnt_mV)  "<GcLDP_ChrgPosHsdCrnt_mV>"
  Bus Selector2/3 -> CCD_DCPosDrvDiag/3(GcLDP_ChrgPosHsdVolt_mV)  "<GcLDP_ChrgPosHsdVolt_mV>"
  Bus Selector2/4 -> CCD_DCPosDrvDiag/4(GcISP_ChrgPosLsdDiag_numb)  "<GcISP_ChrgPosLsdDiag_numb>"
  Bus Selector2/5 -> CCD_DCPosDrvDiag/5(GbCTC_DCPosChrgCtlState_flg)  "<GbCTC_DCPosChrgCtlState_flg>"
  Bus Selector2/6 -> CCD_DCPosDrvDiag/6(GbLDP_ChrgPosHsdCrntVld_flg)  "<GbLDP_ChrgPosHsdCrntVld_flg>"
  Bus Selector2/7 -> CCD_DCPosDrvDiag/7(GbLDP_ChrgPosHsdVoltVld_flg)  "<GbLDP_ChrgPosHsdVoltVld_flg>"
  CCD_DCPosDrvDiag/1(GbCCD_DCPosDrvSTV_flg) -> GbCCD_DCPosDrvSTV_flg/1
  CCD_DCPosDrvDiag/2(GbCCD_DCPosDrvSTG_flg) -> GbCCD_DCPosDrvSTG_flg/1
  CCD_DCPosDrvDiag/3(GbCCD_DCPosDrvOpen_flg) -> GbCCD_DCPosDrvOpen_flg/1
  CCD_DCNegDrvDiag/1(GbCCD_DCNegDrvSTV_flg) -> GbCCD_DCNegDrvSTV_flg/1
  CCD_DCNegDrvDiag/2(GbCCD_DCNegDrvSTG_flg) -> GbCCD_DCNegDrvSTG_flg/1
  CCD_DCNegDrvDiag/3(GbCCD_DCNegDrvOpen_flg) -> GbCCD_DCNegDrvOpen_flg/1
  GcLDP_ChrgNegHsdCrnt_mV/1 -> Bus Creator/25
  Bus Selector3/1 -> CCD_DCNegDrvDiag/1(LbCCD_CCDDiag_flg)  "<LbCCD_CCDDiag_flg>"
  Bus Selector3/2 -> CCD_DCNegDrvDiag/2(GcLDP_ChrgNegHsdCrnt_mV)  "<GcLDP_ChrgNegHsdCrnt_mV>"
  Bus Selector3/3 -> CCD_DCNegDrvDiag/3(GcLDP_ChrgNegHsdVolt_mV)  "<GcLDP_ChrgNegHsdVolt_mV>"
  Bus Selector3/4 -> CCD_DCNegDrvDiag/4(GcISP_ChrgNegLsdDiag_numb)  "<GcISP_ChrgNegLsdDiag_numb>"
  Bus Selector3/5 -> CCD_DCNegDrvDiag/5(GbCTC_DCNegChrgCtlState_flg)  "<GbCTC_DCNegChrgCtlState_flg>"
  Bus Selector3/6 -> CCD_DCNegDrvDiag/6(GbLDP_ChrgNegHsdCrntVld_flg)  "<GbLDP_ChrgNegHsdCrntVld_flg>"
  Bus Selector3/7 -> CCD_DCNegDrvDiag/7(GbLDP_ChrgNegHsdVoltVld_flg)  "<GbLDP_ChrgNegHsdVoltVld_flg>"
  CCD_MPosDrvDiag/4(GbCCD_PosDrvFlt_flg) -> GbCCD_PosgDrvFlt_flg/1
  CCD_MNegDrvDiag/4(GbCCD_NegDrvFlt_flg) -> GbCCD_NegDrvFlt_flg/1
  CCD_DCPosDrvDiag/4(GbCCD_DCPosDrvFlt_flg) -> GbCCD_DCPosDrvFlt_flg/1
  CCD_DCNegDrvDiag/4(GbCCD_DCNegDrvFlt_flg) -> GbCCD_DCNegDrvFlt_flg/1
  GeUDS_AreaSel_enum/1 -> Bus Creator/26
  Bus Selector4/1 -> Data Type Conversion1/1  "<GeUDS_AreaSel_enum>"
  Comparison4/1 -> CCD_DCPosDrvDiag/Enable
  Constant1/1 -> Comparison4/2
  Data Type Conversion1/1 -> Comparison4/1

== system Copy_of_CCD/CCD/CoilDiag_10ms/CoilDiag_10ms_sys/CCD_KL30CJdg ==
  GcLDP_Kl30Volt_mV : Inport
  Constant1 : Constant  Value=CcCCD_KL30CVoltHiLmt_mV
  Constant2 : Constant  Value=CCD_RUNTIME_MS
  Constant3 : Constant  Value=CcCCD_KL30CVoltCnf_ms
  Constant4 : Constant  Value=CcCCD_KL30CVoltLoLmt_mV
  Delay : AIWAYS_Powertrain_BMS_lib/Debounce & Delay/BMSDelay
  LbCCD_CCDDiag_flgOverWrite : AIWAYS_Powertrain_BMS_lib/Signals/OverWrite  OverWrite_Value=CbCCD_CCDDiagOvr_flg  OverWrite_flag=CbCCD_CCDDiagOvrSwt_flg
  Logical Operator5 : Logic  AllPortsSameDT=off  OutDataTypeStr=boolean
  Relational Operator1 : RelationalOperator  OutDataTypeStr=boolean
  Relational Operator6 : RelationalOperator  Operator=<=  OutDataTypeStr=boolean
  LbCCD_CCDDiag_flg : Outport
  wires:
  Delay/1 -> LbCCD_CCDDiag_flgOverWrite/1
  Logical Operator5/1 -> Delay/1
  Constant4/1 -> Relational Operator1/2
  Relational Operator6/1 -> Logical Operator5/2
  Relational Operator1/1 -> Logical Operator5/1
  Constant3/1 -> Delay/3
  Constant1/1 -> Relational Operator6/2
  Constant2/1 -> Delay/2
  GcLDP_Kl30Volt_mV/1 -> Relational Operator1/1, Relational Operator6/1
  LbCCD_CCDDiag_flgOverWrite/1 -> LbCCD_CCDDiag_flg/1  "LbCCD_CCDDiag_flg"

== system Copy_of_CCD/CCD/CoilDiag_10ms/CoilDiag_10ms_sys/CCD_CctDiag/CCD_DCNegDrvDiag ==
  LbCCD_CCDDiag_flg : Inport
  GcLDP_ChrgNegHsdCrnt_mV : Inport  Port=2
  GcLDP_ChrgNegHsdVolt_mV : Inport  Port=3
  GcISP_ChrgNegLsdDiag_numb : Inport  Port=4
  GbCTC_DCNegChrgCtlState_flg : Inport  Port=5
  GbLDP_ChrgNegHsdCrntVld_flg : Inport  Port=6
  GbLDP_ChrgNegHsdVoltVld_flg : Inport  Port=7
  Bus Creator : BusCreator  Inputs=7
  Bus Selector{1..4} (4 alike) : BusSelector  OutputSignals=LbCCD_CCDDiag_flg,GcLDP_ChrgNegHsdVolt_mV,GcISP_ChrgNegLsdDiag_numb,GbCTC_DCNegChrgCtlState_flg,GbLDP_ChrgNegHsdVoltVld_flg
  CCD_DCNegDrvFlt : Subsystem
  CCD_DCNegDrvOpenDiag : Subsystem
  CCD_DCNegDrvSTGDiag : Subsystem
  CCD_DCNegDrvSTVDiag : Subsystem
  GbCCD_DCNegDrvSTV_flg : Outport
  GbCCD_DCNegDrvSTG_flg : Outport  Port=2
  GbCCD_DCNegDrvOpen_flg : Outport  Port=3
  GbCCD_DCNegDrvFlt_flg : Outport  Port=4
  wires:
  LbCCD_CCDDiag_flg/1 -> Bus Creator/1
  GcLDP_ChrgNegHsdCrnt_mV/1 -> Bus Creator/2
  GcLDP_ChrgNegHsdVolt_mV/1 -> Bus Creator/3
  GcISP_ChrgNegLsdDiag_numb/1 -> Bus Creator/4
  GbCTC_DCNegChrgCtlState_flg/1 -> Bus Creator/5
  GbLDP_ChrgNegHsdCrntVld_flg/1 -> Bus Creator/6
  GbLDP_ChrgNegHsdVoltVld_flg/1 -> Bus Creator/7
  Bus Creator/1 -> Bus Selector4/1, Bus Selector3/1, Bus Selector2/1, Bus Selector1/1
  CCD_DCNegDrvSTVDiag/1(GbCCD_DCNegDrvSTV_flg) -> GbCCD_DCNegDrvSTV_flg/1
  Bus Selector1/1 -> CCD_DCNegDrvSTVDiag/1(LbCCD_CCDDiag_flg)  "<LbCCD_CCDDiag_flg>"
  Bus Selector1/2 -> CCD_DCNegDrvSTVDiag/2(GcLDP_ChrgNegHsdVolt_mV)  "<GcLDP_ChrgNegHsdVolt_mV>"
  Bus Selector1/3 -> CCD_DCNegDrvSTVDiag/3(GcISP_ChrgNegLsdDiag_numb)  "<GcISP_ChrgNegLsdDiag_numb>"
  Bus Selector1/4 -> CCD_DCNegDrvSTVDiag/4(GbCTC_DCNegChrgCtlState_flg)  "<GbCTC_DCNegChrgCtlState_flg>"
  Bus Selector1/5 -> CCD_DCNegDrvSTVDiag/5(GbLDP_ChrgNegHsdVoltVld_flg)  "<GbLDP_ChrgNegHsdVoltVld_flg>"
  Bus Selector2/2 -> CCD_DCNegDrvSTGDiag/2(GcLDP_ChrgNegHsdVolt_mV)  "<GcLDP_ChrgNegHsdVolt_mV>"
  Bus Selector2/1 -> CCD_DCNegDrvSTGDiag/1(LbCCD_CCDDiag_flg)  "<LbCCD_CCDDiag_flg>"
  Bus Selector2/3 -> CCD_DCNegDrvSTGDiag/3(GcISP_ChrgNegLsdDiag_numb)  "<GcISP_ChrgNegLsdDiag_numb>"
  Bus Selector2/4 -> CCD_DCNegDrvSTGDiag/4(GbCTC_DCNegChrgCtlState_flg)  "<GbCTC_DCNegChrgCtlState_flg>"
  Bus Selector2/5 -> CCD_DCNegDrvSTGDiag/5(GbLDP_ChrgNegHsdVoltVld_flg)  "<GbLDP_ChrgNegHsdVoltVld_flg>"
  Bus Selector3/1 -> CCD_DCNegDrvOpenDiag/1(LbCCD_CCDDiag_flg)  "<LbCCD_CCDDiag_flg>"
  Bus Selector3/2 -> CCD_DCNegDrvOpenDiag/2(GcLDP_ChrgNegHsdVolt_mV)  "<GcLDP_ChrgNegHsdVolt_mV>"
  Bus Selector3/3 -> CCD_DCNegDrvOpenDiag/3(GcISP_ChrgNegLsdDiag_numb)  "<GcISP_ChrgNegLsdDiag_numb>"
  Bus Selector3/4 -> CCD_DCNegDrvOpenDiag/4(GbCTC_DCNegChrgCtlState_flg)  "<GbCTC_DCNegChrgCtlState_flg>"
  Bus Selector3/5 -> CCD_DCNegDrvOpenDiag/5(GbLDP_ChrgNegHsdVoltVld_flg)  "<GbLDP_ChrgNegHsdVoltVld_flg>"
  CCD_DCNegDrvOpenDiag/1(GbCCD_DCNegDrvOpen_flg) -> GbCCD_DCNegDrvOpen_flg/1
  CCD_DCNegDrvSTGDiag/1(GbCCD_DCNegDrvSTG_flg) -> GbCCD_DCNegDrvSTG_flg/1
  CCD_DCNegDrvFlt/1(GbCCD_DCNegDrvFlt_flg) -> GbCCD_DCNegDrvFlt_flg/1
  Bus Selector4/1 -> CCD_DCNegDrvFlt/1(LbCCD_CCDDiag_flg)  "<LbCCD_CCDDiag_flg>"
  Bus Selector4/2 -> CCD_DCNegDrvFlt/2(GcLDP_ChrgNegHsdVolt_mV)  "<GcLDP_ChrgNegHsdVolt_mV>"
  Bus Selector4/3 -> CCD_DCNegDrvFlt/3(GcISP_ChrgNegLsdDiag_numb)  "<GcISP_ChrgNegLsdDiag_numb>"
  Bus Selector4/4 -> CCD_DCNegDrvFlt/4(GbCTC_DCNegChrgCtlState_flg)  "<GbCTC_DCNegChrgCtlState_flg>"
  Bus Selector4/5 -> CCD_DCNegDrvFlt/5(GbLDP_ChrgNegHsdVoltVld_flg)  "<GbLDP_ChrgNegHsdVoltVld_flg>"

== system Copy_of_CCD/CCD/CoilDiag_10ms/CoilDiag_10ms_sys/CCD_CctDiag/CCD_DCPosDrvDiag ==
  LbCCD_CCDDiag_flg : Inport
  GcLDP_ChrgPosHsdCrnt_mV : Inport  Port=2
  GcLDP_ChrgPosHsdVolt_mV : Inport  Port=3
  GcISP_ChrgPosLsdDiag_numb : Inport  Port=4
  GbCTC_DCPosChrgCtlState_flg : Inport  Port=5
  GbLDP_ChrgPosHsdCrntVld_flg : Inport  Port=6
  GbLDP_ChrgPosHsdVoltVld_flg : Inport  Port=7
  Enable : EnablePort  StatesWhenEnabling=reset
  Bus Creator : BusCreator  Inputs=7
  Bus Selector{1..4} (4 alike) : BusSelector  OutputSignals=LbCCD_CCDDiag_flg,GcLDP_ChrgPosHsdVolt_mV,GcISP_ChrgPosLsdDiag_numb,GbCTC_DCPosChrgCtlState_flg,GbLDP_ChrgPosHsdVoltVld_flg
  CCD_DCPosDrvFlt : Subsystem
  CCD_DCPosDrvOpenDiag : Subsystem
  CCD_DCPosDrvSTGDiag : Subsystem
  CCD_DCPosDrvSTVDiag : Subsystem
  GbCCD_DCPosDrvSTV_flg : Outport
  GbCCD_DCPosDrvSTG_flg : Outport  Port=2
  GbCCD_DCPosDrvOpen_flg : Outport  Port=3
  GbCCD_DCPosDrvFlt_flg : Outport  Port=4
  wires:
  CCD_DCPosDrvSTGDiag/1(GbCCD_DCPosDrvSTG_flg) -> GbCCD_DCPosDrvSTG_flg/1
  CCD_DCPosDrvOpenDiag/1(GbCCD_DCPosDrvOpen_flg) -> GbCCD_DCPosDrvOpen_flg/1
  Bus Selector1/5 -> CCD_DCPosDrvSTVDiag/5(GbLDP_ChrgPosHsdVoltVld_flg)  "<GbLDP_ChrgPosHsdVoltVld_flg>"
  Bus Selector1/4 -> CCD_DCPosDrvSTVDiag/4(GbCTC_DCPosChrgCtlState_flg)  "<GbCTC_DCPosChrgCtlState_flg>"
  Bus Selector1/3 -> CCD_DCPosDrvSTVDiag/3(GcISP_ChrgPosLsdDiag_numb)  "<GcISP_ChrgPosLsdDiag_numb>"
  Bus Selector1/2 -> CCD_DCPosDrvSTVDiag/2(GcLDP_ChrgPosHsdVolt_mV)  "<GcLDP_ChrgPosHsdVolt_mV>"
  Bus Selector1/1 -> CCD_DCPosDrvSTVDiag/1(LbCCD_CCDDiag_flg)  "<LbCCD_CCDDiag_flg>"
  CCD_DCPosDrvSTVDiag/1(GbCCD_DCPosDrvSTV_flg) -> GbCCD_DCPosDrvSTV_flg/1
  Bus Creator/1 -> Bus Selector1/1, Bus Selector4/1, Bus Selector3/1, Bus Selector2/1
  GbLDP_ChrgPosHsdVoltVld_flg/1 -> Bus Creator/7
  GbLDP_ChrgPosHsdCrntVld_flg/1 -> Bus Creator/6
  GbCTC_DCPosChrgCtlState_flg/1 -> Bus Creator/5
  GcISP_ChrgPosLsdDiag_numb/1 -> Bus Creator/4
  GcLDP_ChrgPosHsdVolt_mV/1 -> Bus Creator/3
  GcLDP_ChrgPosHsdCrnt_mV/1 -> Bus Creator/2
  LbCCD_CCDDiag_flg/1 -> Bus Creator/1
  Bus Selector2/1 -> CCD_DCPosDrvSTGDiag/1(LbCCD_CCDDiag_flg)  "<LbCCD_CCDDiag_flg>"
  Bus Selector2/2 -> CCD_DCPosDrvSTGDiag/2(GcLDP_ChrgPosHsdVolt_mV)  "<GcLDP_ChrgPosHsdVolt_mV>"
  Bus Selector2/3 -> CCD_DCPosDrvSTGDiag/3(GcISP_ChrgPosLsdDiag_numb)  "<GcISP_ChrgPosLsdDiag_numb>"
  Bus Selector2/4 -> CCD_DCPosDrvSTGDiag/4(GbCTC_DCPosChrgCtlState_flg)  "<GbCTC_DCPosChrgCtlState_flg>"
  Bus Selector2/5 -> CCD_DCPosDrvSTGDiag/5(GbLDP_ChrgPosHsdVoltVld_flg)  "<GbLDP_ChrgPosHsdVoltVld_flg>"
  Bus Selector3/1 -> CCD_DCPosDrvOpenDiag/1(LbCCD_CCDDiag_flg)  "<LbCCD_CCDDiag_flg>"
  Bus Selector3/2 -> CCD_DCPosDrvOpenDiag/2(GcLDP_ChrgPosHsdVolt_mV)  "<GcLDP_ChrgPosHsdVolt_mV>"
  Bus Selector3/3 -> CCD_DCPosDrvOpenDiag/3(GcISP_ChrgPosLsdDiag_numb)  "<GcISP_ChrgPosLsdDiag_numb>"
  Bus Selector3/4 -> CCD_DCPosDrvOpenDiag/4(GbCTC_DCPosChrgCtlState_flg)  "<GbCTC_DCPosChrgCtlState_flg>"
  Bus Selector3/5 -> CCD_DCPosDrvOpenDiag/5(GbLDP_ChrgPosHsdVoltVld_flg)  "<GbLDP_ChrgPosHsdVoltVld_flg>"
  CCD_DCPosDrvFlt/1(GbCCD_DCPosDrvFlt_flg) -> GbCCD_DCPosDrvFlt_flg/1
  Bus Selector4/3 -> CCD_DCPosDrvFlt/3(GcISP_ChrgPosLsdDiag_numb)  "<GcISP_ChrgPosLsdDiag_numb>"
  Bus Selector4/1 -> CCD_DCPosDrvFlt/1(LbCCD_CCDDiag_flg)  "<LbCCD_CCDDiag_flg>"
  Bus Selector4/2 -> CCD_DCPosDrvFlt/2(GcLDP_ChrgPosHsdVolt_mV)  "<GcLDP_ChrgPosHsdVolt_mV>"
  Bus Selector4/4 -> CCD_DCPosDrvFlt/4(GbCTC_DCPosChrgCtlState_flg)  "<GbCTC_DCPosChrgCtlState_flg>"
  Bus Selector4/5 -> CCD_DCPosDrvFlt/5(GbLDP_ChrgPosHsdVoltVld_flg)  "<GbLDP_ChrgPosHsdVoltVld_flg>"

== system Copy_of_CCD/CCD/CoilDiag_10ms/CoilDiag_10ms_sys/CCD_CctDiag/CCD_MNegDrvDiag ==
  LbCCD_CCDDiag_flg : Inport
  GcLDP_NegHsdCrnt_mV : Inport  Port=2
  GcLDP_NegHsdVolt_mV : Inport  Port=3
  GcISP_NegLsdDiag_numb : Inport  Port=4
  GbCTC_NegCtlState_flg : Inport  Port=5
  GbLDP_NegHsdCrntVld_flg : Inport  Port=6
  GbLDP_NegHsdVoltVld_flg : Inport  Port=7
  Bus Creator : BusCreator  Inputs=7
  Bus Selector{1..4} (4 alike) : BusSelector  OutputSignals=LbCCD_CCDDiag_flg,GcLDP_NegHsdVolt_mV,GcISP_NegLsdDiag_numb,GbCTC_NegCtlState_flg,GbLDP_NegHsdVoltVld_flg
  CCD_NegDrvFlt : Subsystem
  CCD_NegDrvOpenDiag : Subsystem
  CCD_NegDrvSTGDiag : Subsystem
  CCD_NegDrvSTVDiag : Subsystem
  GbCCD_NegDrvSTV_flg : Outport
  GbCCD_NegDrvSTG_flg : Outport  Port=2
  GbCCD_NegDrvOpen_flg : Outport  Port=3
  GbCCD_NegDrvFlt_flg : Outport  Port=4
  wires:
  CCD_NegDrvSTGDiag/1(GbCCD_NegDrvSTG_flg) -> GbCCD_NegDrvSTG_flg/1
  CCD_NegDrvOpenDiag/1(GbCCD_NegDrvOpen_flg) -> GbCCD_NegDrvOpen_flg/1
  Bus Selector3/5 -> CCD_NegDrvOpenDiag/5(GbLDP_NegHsdVoltVld_flg)  "<GbLDP_NegHsdVoltVld_flg>"
  Bus Selector3/4 -> CCD_NegDrvOpenDiag/4(GbCTC_NegCtlState_flg)  "<GbCTC_NegCtlState_flg>"
  Bus Selector3/3 -> CCD_NegDrvOpenDiag/3(GcISP_NegLsdDiag_numb)  "<GcISP_NegLsdDiag_numb>"
  Bus Selector3/2 -> CCD_NegDrvOpenDiag/2(GcLDP_NegHsdVolt_mV)  "<GcLDP_NegHsdVolt_mV>"
  Bus Selector3/1 -> CCD_NegDrvOpenDiag/1(LbCCD_CCDDiag_flg)  "<LbCCD_CCDDiag_flg>"
  Bus Selector2/5 -> CCD_NegDrvSTGDiag/5(GbLDP_NegHsdVoltVld_flg)  "<GbLDP_NegHsdVoltVld_flg>"
  Bus Selector2/4 -> CCD_NegDrvSTGDiag/4(GbCTC_NegCtlState_flg)  "<GbCTC_NegCtlState_flg>"
  Bus Selector2/3 -> CCD_NegDrvSTGDiag/3(GcISP_NegLsdDiag_numb)  "<GcISP_NegLsdDiag_numb>"
  Bus Selector2/1 -> CCD_NegDrvSTGDiag/1(LbCCD_CCDDiag_flg)  "<LbCCD_CCDDiag_flg>"
  Bus Selector2/2 -> CCD_NegDrvSTGDiag/2(GcLDP_NegHsdVolt_mV)  "<GcLDP_NegHsdVolt_mV>"
  Bus Selector1/5 -> CCD_NegDrvSTVDiag/5(GbLDP_NegHsdVoltVld_flg)  "<GbLDP_NegHsdVoltVld_flg>"
  Bus Selector1/4 -> CCD_NegDrvSTVDiag/4(GbCTC_NegCtlState_flg)  "<GbCTC_NegCtlState_flg>"
  Bus Selector1/3 -> CCD_NegDrvSTVDiag/3(GcISP_NegLsdDiag_numb)  "<GcISP_NegLsdDiag_numb>"
  Bus Selector1/2 -> CCD_NegDrvSTVDiag/2(GcLDP_NegHsdVolt_mV)  "<GcLDP_NegHsdVolt_mV>"
  Bus Selector1/1 -> CCD_NegDrvSTVDiag/1(LbCCD_CCDDiag_flg)  "<LbCCD_CCDDiag_flg>"
  CCD_NegDrvSTVDiag/1(GbCCD_NegDrvSTV_flg) -> GbCCD_NegDrvSTV_flg/1
  Bus Creator/1 -> Bus Selector1/1, Bus Selector3/1, Bus Selector4/1, Bus Selector2/1
  GbLDP_NegHsdVoltVld_flg/1 -> Bus Creator/7
  GbLDP_NegHsdCrntVld_flg/1 -> Bus Creator/6
  GbCTC_NegCtlState_flg/1 -> Bus Creator/5
  GcISP_NegLsdDiag_numb/1 -> Bus Creator/4
  GcLDP_NegHsdVolt_mV/1 -> Bus Creator/3
  GcLDP_NegHsdCrnt_mV/1 -> Bus Creator/2
  LbCCD_CCDDiag_flg/1 -> Bus Creator/1
  CCD_NegDrvFlt/1(GbCCD_NegDrvFlt_flg) -> GbCCD_NegDrvFlt_flg/1
  Bus Selector4/1 -> CCD_NegDrvFlt/1(LbCCD_CCDDiag_flg)  "<LbCCD_CCDDiag_flg>"
  Bus Selector4/2 -> CCD_NegDrvFlt/2(GcLDP_NegHsdVolt_mV)  "<GcLDP_NegHsdVolt_mV>"
  Bus Selector4/3 -> CCD_NegDrvFlt/3(GcISP_NegLsdDiag_numb)  "<GcISP_NegLsdDiag_numb>"
  Bus Selector4/4 -> CCD_NegDrvFlt/4(GbCTC_NegCtlState_flg)  "<GbCTC_NegCtlState_flg>"
  Bus Selector4/5 -> CCD_NegDrvFlt/5(GbLDP_NegHsdVoltVld_flg)  "<GbLDP_NegHsdVoltVld_flg>"

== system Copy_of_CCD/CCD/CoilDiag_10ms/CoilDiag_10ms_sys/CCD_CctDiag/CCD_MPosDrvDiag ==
  LbCCD_CCDDiag_flg : Inport
  GcLDP_PosHsdCrnt_mV : Inport  Port=2
  GcLDP_PosHsdVolt_mV : Inport  Port=3
  GcISP_PosLsdDiag_numb : Inport  Port=4
  GbCTC_PosCtlState_flg : Inport  Port=5
  GbLDP_PosHsdCrntVld_flg : Inport  Port=6
  GbLDP_PosHsdVoltVld_flg : Inport  Port=7
  Bus Creator : BusCreator  Inputs=7
  Bus Selector{1..4} (4 alike) : BusSelector  OutputSignals=LbCCD_CCDDiag_flg,GcLDP_PosHsdVolt_mV,GcISP_PosLsdDiag_numb,GbCTC_PosCtlState_flg,GbLDP_PosHsdVoltVld_flg
  CCD_PosDrvFlt : Subsystem
  CCD_PosDrvOpenDiag : Subsystem
  CCD_PosDrvSTGDiag : Subsystem
  CCD_PosDrvSTVDiag : Subsystem
  GbCCD_PosDrvSTV_flg : Outport
  GbCCD_PosDrvSTG_flg : Outport  Port=2
  GbCCD_PosDrvOpen_flg : Outport  Port=3
  GbCCD_PosDrvFlt_flg : Outport  Port=4
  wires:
  LbCCD_CCDDiag_flg/1 -> Bus Creator/1
  GcLDP_PosHsdCrnt_mV/1 -> Bus Creator/2
  GcLDP_PosHsdVolt_mV/1 -> Bus Creator/3
  GcISP_PosLsdDiag_numb/1 -> Bus Creator/4
  GbCTC_PosCtlState_flg/1 -> Bus Creator/5
  GbLDP_PosHsdCrntVld_flg/1 -> Bus Creator/6
  GbLDP_PosHsdVoltVld_flg/1 -> Bus Creator/7
  Bus Creator/1 -> Bus Selector4/1, Bus Selector3/1, Bus Selector2/1, Bus Selector1/1
  CCD_PosDrvSTVDiag/1(GbCCD_PosDrvSTV_flg) -> GbCCD_PosDrvSTV_flg/1
  Bus Selector1/1 -> CCD_PosDrvSTVDiag/1(LbCCD_CCDDiag_flg)  "<LbCCD_CCDDiag_flg>"
  Bus Selector1/2 -> CCD_PosDrvSTVDiag/2(GcLDP_PosHsdVolt_mV)  "<GcLDP_PosHsdVolt_mV>"
  Bus Selector1/3 -> CCD_PosDrvSTVDiag/3(GcISP_PosLsdDiag_numb)  "<GcISP_PosLsdDiag_numb>"
  Bus Selector1/4 -> CCD_PosDrvSTVDiag/4(GbCTC_PosCtlState_flg)  "<GbCTC_PosCtlState_flg>"
  Bus Selector1/5 -> CCD_PosDrvSTVDiag/5(GbLDP_PosHsdVoltVld_flg)  "<GbLDP_PosHsdVoltVld_flg>"
  Bus Selector2/2 -> CCD_PosDrvSTGDiag/2(GcLDP_PosHsdVolt_mV)  "<GcLDP_PosHsdVolt_mV>"
  Bus Selector2/1 -> CCD_PosDrvSTGDiag/1(LbCCD_CCDDiag_flg)  "<LbCCD_CCDDiag_flg>"
  Bus Selector2/3 -> CCD_PosDrvSTGDiag/3(GcISP_PosLsdDiag_numb)  "<GcISP_PosLsdDiag_numb>"
  Bus Selector2/4 -> CCD_PosDrvSTGDiag/4(GbCTC_PosCtlState_flg)  "<GbCTC_PosCtlState_flg>"
  Bus Selector2/5 -> CCD_PosDrvSTGDiag/5(GbLDP_PosHsdVoltVld_flg)  "<GbLDP_PosHsdVoltVld_flg>"
  Bus Selector3/1 -> CCD_PosDrvOpenDiag/1(LbCCD_CCDDiag_flg)  "<LbCCD_CCDDiag_flg>"
  Bus Selector3/2 -> CCD_PosDrvOpenDiag/2(GcLDP_PosHsdVolt_mV)  "<GcLDP_PosHsdVolt_mV>"
  Bus Selector3/3 -> CCD_PosDrvOpenDiag/3(GcISP_PosLsdDiag_numb)  "<GcISP_PosLsdDiag_numb>"
  Bus Selector3/4 -> CCD_PosDrvOpenDiag/4(GbCTC_PosCtlState_flg)  "<GbCTC_PosCtlState_flg>"
  Bus Selector3/5 -> CCD_PosDrvOpenDiag/5(GbLDP_PosHsdVoltVld_flg)  "<GbLDP_PosHsdVoltVld_flg>"
  CCD_PosDrvOpenDiag/1(GbCCD_PosDrvOpen_flg) -> GbCCD_PosDrvOpen_flg/1
  CCD_PosDrvSTGDiag/1(GbCCD_PosDrvSTG_flg) -> GbCCD_PosDrvSTG_flg/1
  CCD_PosDrvFlt/1(GbCCD_PosDrvFlt_flg) -> GbCCD_PosDrvFlt_flg/1
  Bus Selector4/1 -> CCD_PosDrvFlt/1(LbCCD_CCDDiag_flg)  "<LbCCD_CCDDiag_flg>"
  Bus Selector4/2 -> CCD_PosDrvFlt/2(GcLDP_PosHsdVolt_mV)  "<GcLDP_PosHsdVolt_mV>"
  Bus Selector4/3 -> CCD_PosDrvFlt/3(GcISP_PosLsdDiag_numb)  "<GcISP_PosLsdDiag_numb>"
  Bus Selector4/4 -> CCD_PosDrvFlt/4(GbCTC_PosCtlState_flg)  "<GbCTC_PosCtlState_flg>"
  Bus Selector4/5 -> CCD_PosDrvFlt/5(GbLDP_PosHsdVoltVld_flg)  "<GbLDP_PosHsdVoltVld_flg>"

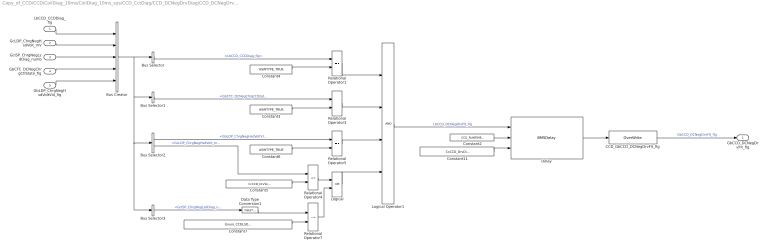
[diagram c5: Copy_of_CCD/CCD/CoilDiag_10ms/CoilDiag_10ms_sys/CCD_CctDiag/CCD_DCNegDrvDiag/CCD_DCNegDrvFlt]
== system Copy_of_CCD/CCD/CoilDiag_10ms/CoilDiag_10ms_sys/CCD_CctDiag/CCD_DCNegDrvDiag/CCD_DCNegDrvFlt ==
  LbCCD_CCDDiag_flg : Inport
  GcLDP_ChrgNegHsdVolt_mV : Inport  Port=2
  GcISP_ChrgNegLsdDiag_numb : Inport  Port=3
  GbCTC_DCNegChrgCtlState_flg : Inport  Port=4
  GbLDP_ChrgNegHsdVoltVld_flg : Inport  Port=5
  Bus Creator : BusCreator  Inputs=5
  Bus Selector : BusSelector  OutputSignals=LbCCD_CCDDiag_flg
  Bus Selector1 : BusSelector  OutputSignals=GbCTC_DCNegChrgCtlState_flg
  Bus Selector2 : BusSelector  OutputSignals=GbLDP_ChrgNegHsdVoltVld_flg,GcLDP_ChrgNegHsdVolt_mV
  Bus Selector3 : BusSelector  OutputSignals=GcISP_ChrgNegLsdDiag_numb
  CCD_GbCCD_DCNegDrvFlt_flg : AIWAYS_Powertrain_BMS_lib/Signals/OverWrite  OverWrite_Value=CbCCD_DCNegDrvFltOvr_flg  OverWrite_flag=CbCCD_DCNegDrvFltOvrSwt_flg
  Constant11 : Constant  Value=CcCCD_DrvDiagtCnf_ms
  Constant2 : Constant  Value=CCD_RUNTIME_MS
  Constant3 : Constant  Value=ASWTYPE_TRUE
  Constant4 : Constant  Value=ASWTYPE_TRUE
  Constant5 : Constant  Value=CcCCD_DrvVoltHiVal_mV
  Constant6 : Constant  Value=ASWTYPE_TRUE
  Constant7 : Constant  Value=Enum_CCDLSDState.Enum_CCDLSDState_OK
  Data Type Conversion1 : DataTypeConversion
  Delay : AIWAYS_Powertrain_BMS_lib/Debounce & Delay/BMSDelay
  Logical : Logic  Operator=OR  OutDataTypeStr=boolean
  Logical Operator1 : Logic  Inputs=4  AllPortsSameDT=off  OutDataTypeStr=boolean
  Relational Operator1 : RelationalOperator  Operator===  OutDataTypeStr=boolean
  Relational Operator3 : RelationalOperator  Operator===  OutDataTypeStr=boolean
  Relational Operator4 : RelationalOperator  Operator=<=  OutDataTypeStr=boolean
  Relational Operator5 : RelationalOperator  Operator===  OutDataTypeStr=boolean
  Relational Operator7 : RelationalOperator  Operator=~=  OutDataTypeStr=boolean
  GbCCD_DCNegDrvFlt_flg : Outport
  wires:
  Constant4/1 -> Relational Operator1/2
  Constant5/1 -> Relational Operator4/2
  Relational Operator1/1 -> Logical Operator1/1
  Constant3/1 -> Relational Operator3/2
  Relational Operator5/1 -> Logical Operator1/3
  Constant7/1 -> Relational Operator7/2
  Bus Selector3/1 -> Data Type Conversion1/1  "<GcISP_ChrgNegLsdDiag_numb>"
  Constant6/1 -> Relational Operator5/2
  Relational Operator3/1 -> Logical Operator1/2
  Data Type Conversion1/1 -> Relational Operator7/1
  Bus Selector2/1 -> Relational Operator5/1  "<GbLDP_ChrgNegHsdVoltVld_flg>"
  Bus Selector2/2 -> Relational Operator4/1  "<GcLDP_ChrgNegHsdVolt_mV>"
  Bus Selector/1 -> Relational Operator1/1  "<LbCCD_CCDDiag_flg>"
  Logical Operator1/1 -> Delay/1  "LbCCD_DCNegDrvFlt_flg"
  Bus Selector1/1 -> Relational Operator3/1  "<GbCTC_DCNegChrgCtlState_flg>"
  Constant2/1 -> Delay/2
  Constant11/1 -> Delay/3
  Delay/1 -> CCD_GbCCD_DCNegDrvFlt_flg/1
  Relational Operator7/1 -> Logical/2
  Relational Operator4/1 -> Logical/1
  Logical/1 -> Logical Operator1/4
  CCD_GbCCD_DCNegDrvFlt_flg/1 -> GbCCD_DCNegDrvFlt_flg/1  "GbCCD_DCNegDrvFlt_flg"
  LbCCD_CCDDiag_flg/1 -> Bus Creator/1
  GcLDP_ChrgNegHsdVolt_mV/1 -> Bus Creator/2
  GcISP_ChrgNegLsdDiag_numb/1 -> Bus Creator/3
  GbLDP_ChrgNegHsdVoltVld_flg/1 -> Bus Creator/5
  GbCTC_DCNegChrgCtlState_flg/1 -> Bus Creator/4
  Bus Creator/1 -> Bus Selector3/1, Bus Selector2/1, Bus Selector1/1, Bus Selector/1
